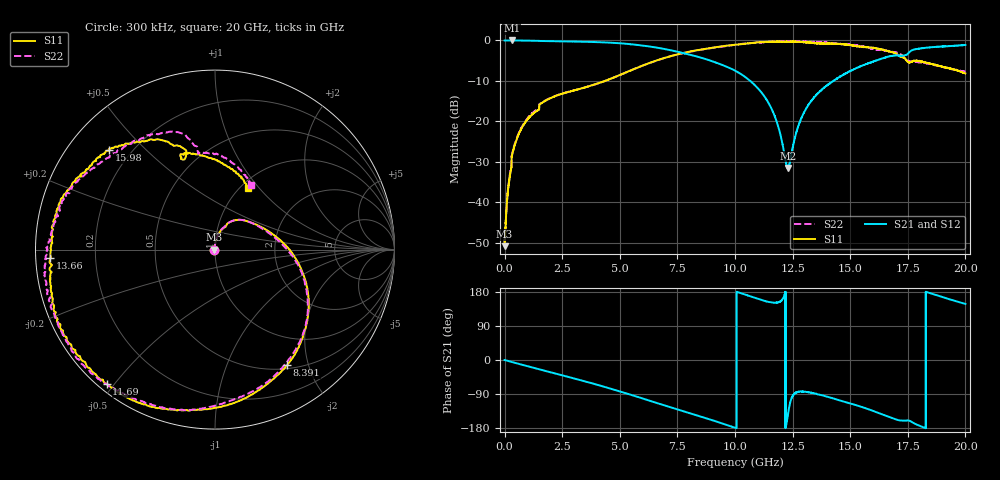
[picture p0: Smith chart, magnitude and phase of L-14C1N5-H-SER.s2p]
!{L-14C1N5}
!Johanson Technology Inc.
!www.johansontechnology.com
!Test Board Conditions:
!Substrate Type  RO4350B
!Substrate Thickness  20 mil
!Substrate Dk  3.66
!TL Type: GCPW
!TL Trace Width  36 mil
!TL Gap  12 mil
!Electrode orientation  Horizontal
!DUT TOPOLOGY	SERIES
!Mounting Pad LxW  26x36 mil
! Created Sun Jun 20 12:53:39 2021
# hz S ma R 50
! 2 Port Network Data from SP1.SP block
! freq  magS11  angS11  magS21  angS21  magS12  angS12  magS22  angS22
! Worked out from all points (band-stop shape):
!   20001 points, 300 kHz to 20 GHz, reference 50 ohm
!   highest |S21| = -0.02 dB at 308.3 MHz (marker M1); lowest = -31.5 dB at 12.29 GHz (marker M2)
!   |S21| within 3 dB of the highest: start of sweep to 7.654 GHz; 17.55 GHz to end of sweep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
!   lowest |S11| = -50.8 dB at 300 kHz (marker M3), VSWR 1.01, Z = 49.7 + j0.019 ohm
!   |S11| at or under -10 dB: start of sweep to 4.368 GHz; 4.36873 GHz to 4.370102 GHz (1.373 MHz wide, 0.0314 % of centre); 4.370552 GHz to 4.371462 GHz (909.9 kHz wide, 0.0208 % of centre)
!   |S22| runs from -50.0 to -0.2 dB; largest |S21 - S12| = 0.02
!   S11 on the Smith chart (normalised r, x): 300 kHz: 0.99, +0.00; 8.391 GHz: 0.55, -1.66; 11.69 GHz: 0.02, -0.48; 13.66 GHz: 0.04, -0.02; 15.98 GHz: 0.12, +0.39; 20 GHz: 1.08, +0.88
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300000  0.002876 176.2  0.9972 -0.1  0.9968 -0.0  0.003173 173.5
1.553e8  0.01471 97.4  0.9978 -2.5  0.9966 -2.5  0.01545 97.4
3.083e8  0.03661 88.0  0.9981 -5.2  0.9961 -5.2  0.03739 87.6
7.023e8  0.07883 79.0  0.9956 -11.6  0.9953 -11.6  0.08068 79.2
1.6003e9  0.1676 63.1  0.9833 -26.3  0.9827 -26.2  0.1696 62.8
3.3343e9  0.2548 35.5  0.9633 -53.9  0.9632 -53.9  0.2554 35.0
5.0343e9  0.3768 6.4  0.9203 -83.6  0.9182 -83.6  0.3763 4.2
6.6673e9  0.5737 -25.3  0.8088 -114.7  0.8055 -114.5  0.5728 -26.4
8.3913e9  0.7593 -58.1  0.6266 -147.0  0.6231 -146.8  0.7555 -59.9
1.00003e10  0.8828 -90.2  0.4233 -178.5  0.4243 -178.3  0.8818 -93.1
1.09913e10  0.9452 -112.4  0.2563 161.6  0.26 161.8  0.9375 -115.2
1.16873e10  0.9621 -128.8  0.1232 151.3  0.1238 151.3  0.9701 -133.1
1.22863e10  0.9625 -144.6  0.0265 -148.9  0.02697 -149.5  0.9714 -147.5
1.27973e10  0.9624 -156.8  0.09556 -83.4  0.09693 -83.9  0.9616 -159.1
1.33343e10  0.9345 -169.5  0.1827 -86.7  0.1824 -87.6  0.9603 -169.6
1.36563e10  0.9191 -177.1  0.2312 -91.3  0.2286 -92.4  0.9515 -175.0
1.49873e10  0.8758 156.1  0.4166 -114.4  0.4111 -114.1  0.889 161.0
1.59773e10  0.8113 136.8  0.5462 -134.0  0.545 -134.1  0.7885 139.8
1.66673e10  0.7313 125.1  0.6328 -149.6  0.6316 -148.0  0.7423 121.3
1.76053e10  0.5373 110.3  0.7305 -161.1  0.7321 -160.9  0.5445 99.8
1.82483e10  0.5379 99.6  0.8081 -179.2  0.8139 -178.7  0.5252 87.1
2e10  0.3904 62.0  0.8779 148.0  0.8782 148.4  0.4089 60.6
